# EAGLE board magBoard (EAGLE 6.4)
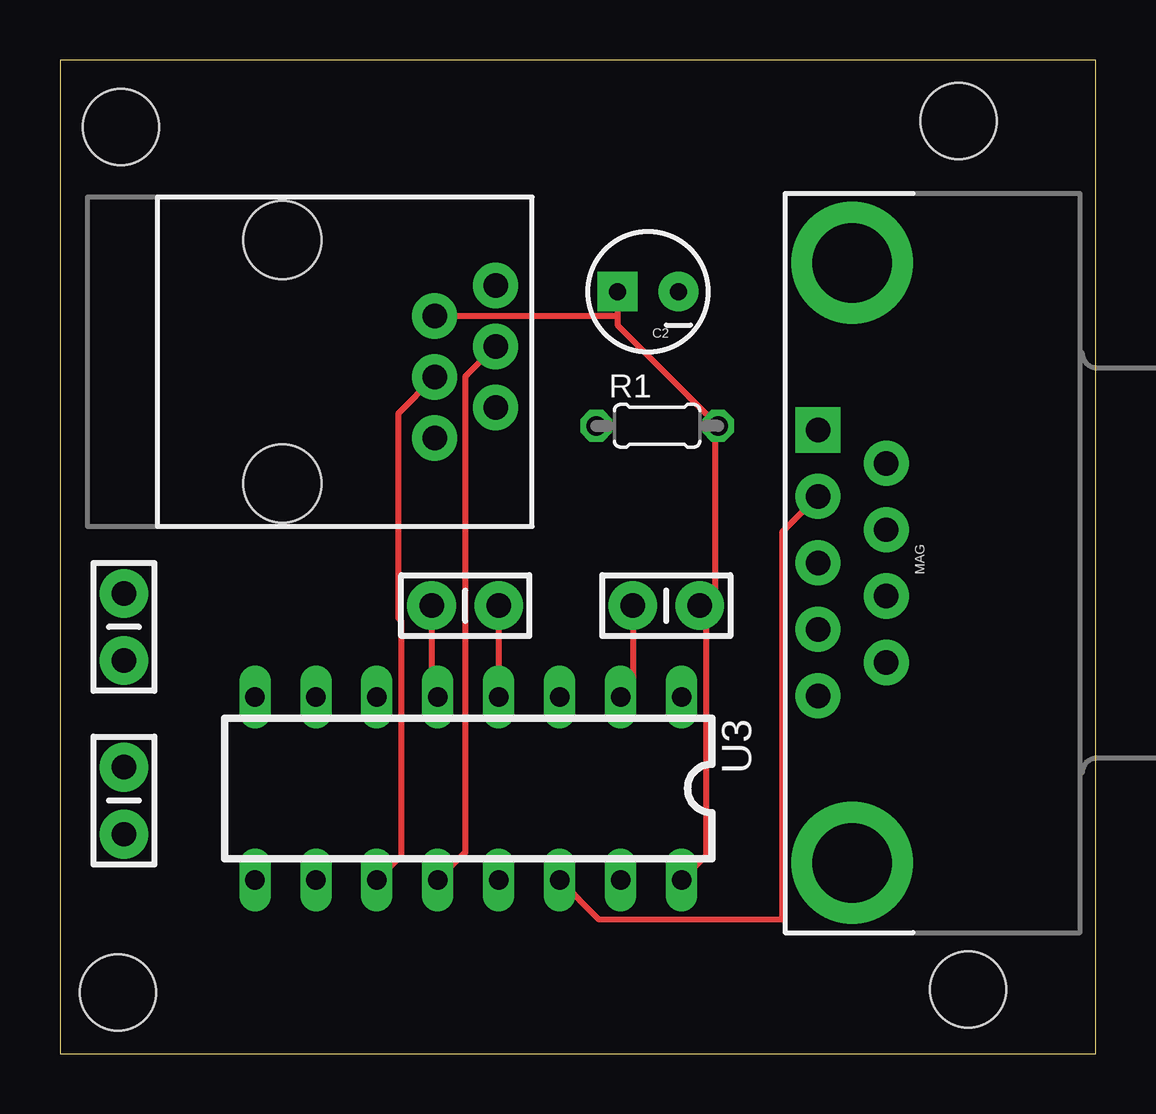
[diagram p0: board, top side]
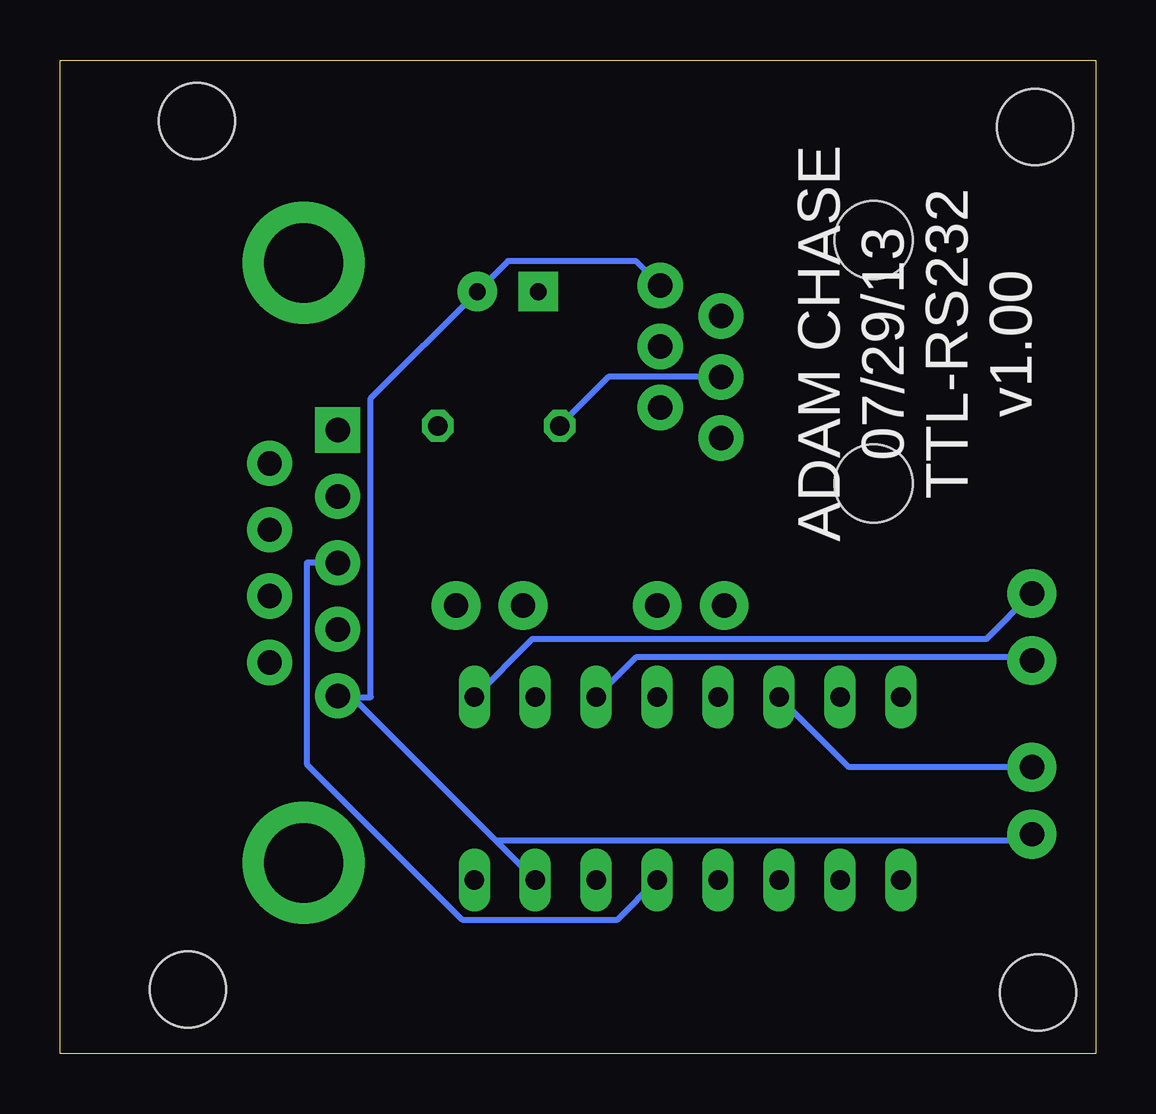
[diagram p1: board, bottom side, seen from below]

Size 43.18 x 41.4 mm. Coordinates in mm from the lower left corner, seen from the top.
Outline: 0,0 43.18,0 43.18,41.4 0,41.39 0,0
Copper layers (1*16): Top 0.035mm / dielectric 1.5mm / Bottom 0.035mm
Design rules "default": minimum track width 10mil, minimum drill 24mil, track to track 8mil, track to pad 8mil, pad to pad 8mil, via to via 8mil, smd to smd 8mil, copper to edge 40mil, drill to drill 8mil, minimum pad ring 10mil, minimum via ring 8mil, stop-mask expansion 4mil, vias tented up to drill 0mil, thermal gap 10mil
Holes 3.17 mm at 2.54,38.61 2.41,2.54 37.85,2.67 37.47,38.86

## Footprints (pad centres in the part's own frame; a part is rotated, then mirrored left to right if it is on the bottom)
CPOL-RADIAL-10UF-25V = drill 0.7 pad 1.651 square: 1 1.27,0 | drill 0.7 pad 1.651: 2 -1.27,0
CAP-PTH-SMALL-KIT = drill 1.016 pad 2.032: 1 -1.397,0; 2 1.397,0
RJ11-6 = drill 1.016 pad 1.88: 1 1.905,8.89; 2 3.175,6.35; 3 4.445,8.89; 4 5.715,6.35; 5 6.985,8.89; 6 8.255,6.35 | hole 3.251: 0,0; 10.16,0
DB9 = drill 1.016 pad 1.88 square: 1 -5.54,-1.42 | drill 1.016 pad 1.88: 2 -2.77,-1.42; 3 0,-1.42; 4 2.77,-1.42; 5 5.54,-1.42; 6 -4.15,1.42; 7 -1.38,1.42; 8 1.38,1.42; 9 4.15,1.42 | drill 3.302 pad 5.08: G1 -12.5,0; G2 12.5,0
0204/5 = drill 0.813 octagon: 1 -2.54,0; 2 2.54,0
DIL16 = drill 0.813 long: 1 -8.89,-3.81; 2 -6.35,-3.81; 3 -3.81,-3.81; 4 -1.27,-3.81; 5 1.27,-3.81; 6 3.81,-3.81; 7 6.35,-3.81; 8 8.89,-3.81; 9 8.89,3.81; 10 6.35,3.81; 11 3.81,3.81; 12 1.27,3.81; 13 -1.27,3.81; 14 -3.81,3.81; 15 -6.35,3.81; 16 -8.89,3.81

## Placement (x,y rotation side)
C2  10uF  [CPOL-RADIAL-10UF-25V]  24.51,31.75 180 top
C3  100nF  [CAP-PTH-SMALL-KIT]  2.67,17.78 270 top
C4  100nF  [CAP-PTH-SMALL-KIT]  25.27,18.67 180 top
C5  100nF  [CAP-PTH-SMALL-KIT]  16.89,18.67 180 top
C6  100nF  [CAP-PTH-SMALL-KIT]  2.67,10.54 270 top
J1  RJ11-6PTH  [RJ11-6]  9.27,33.91 270 top
MAG  RS232  [DB9]  33.02,20.45 270 top
R1  1K  [0204/5]  24.89,26.16 0 top
U3  MAX232PTH  [DIL16]  17.02,11.05 180 top

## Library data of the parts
C2-C6 = SparkFun-Capacitors
J1 MAG = SparkFun-Connectors
R1 = rcl
U3 = SparkFun-DigitalIC

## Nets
GND: C2.2 C6.2 J1.1 MAG.5 U3.15
N$2: C3.1 U3.1
N$3: C3.2 U3.3
N$4: C5.1 U3.4
N$5: C5.2 U3.5
N$8: C4.2 U3.2
N$12: C6.1 U3.6
N$16: MAG.3 U3.13
N$17: MAG.2 U3.14
RX: J1.3 U3.12
TX: J1.4 R1.1 U3.11
VH: C2.1 C4.1 J1.2 R1.2 U3.16

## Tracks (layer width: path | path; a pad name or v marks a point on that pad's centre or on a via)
GND
  Bottom 0.254: J1.1 19.18,33.02 24.51,33.02 C2.2 30.23,27.3 30.23,14.86 30.86,14.86 MAG.5 31.5,14.86 30.99,14.86 24.96,8.83 | 24.96,8.83 U3.15 | C6.2 2.92,8.89 24.89,8.89 24.96,8.83
N$2
  Bottom 0.254: U3.1 23.5,17.27 4.57,17.27 C3.1
N$3
  Bottom 0.254: U3.3 19.18,16.51 2.79,16.51 C3.2
N$4
  Top 0.254: C5.1 U3.4
N$5
  Top 0.254: U3.5 15.49,15.11 C5.2
N$8
  Top 0.254: U3.2 23.88,15.37 C4.2
N$12
  Bottom 0.254: U3.6 10.29,11.94 C6.1
N$16
  Bottom 0.254: U3.13 19.94,5.59 26.42,5.59 32.89,12.06 32.89,20.45 MAG.3
N$17
  Top 0.254: U3.14 22.48,5.59 30.1,5.59 30.1,21.72 31.5,23.11 MAG.2
RX
  Top 0.254: U3.12 16.89,8.38 16.89,28.19 J1.3
TX
  Top 0.254: U3.11 14.22,8.26 14.22,18.03 14.1,18.16 14.1,26.67 J1.4
  Bottom 0.254: R1.1 20.32,28.19 J1.4
VH
  Top 0.254: U3.16 26.92,8.26 26.92,18.41 C4.1 26.8,18.67 27.3,19.18 27.3,26.16 R1.2 23.24,30.35 23.24,30.73 | C2.1 23.24,30.73 | 23.24,30.73 J1.2

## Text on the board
bPlace: ADAM CHASE / 07/29/13 / TTL-RS232 / v1.00

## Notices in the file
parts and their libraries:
SparkFun-Capacitors: Licensing: CC v3.0 Share-Alike You are welcome to use this library for commercial purposes.
